[IBIS Ver]   3.2
[File Name]   sprm456.ibs
[File Rev]   1.0
[Date]   November 3, 2003
[Source]   File originated at Texas Instruments
[Copyright]   (c) 2003, Texas Instruments Inc.
[Component]   r2812pgf
[Manufacturer] Texas Instruments
[Package]
| Variable   Typ   Min   Max
R_pkg   0.198   0.1909   0.2047
L_pkg   8.904e-09   8.346e-09   9.905e-09
C_pkg   1.561e-12   1.156e-12   1.834e-12
[Pin] signal_name   model_name   R_pin   L_pin   C_pin
1   VDDAIO   NC   0.1921  9.905e-09  1.489e-12
2   ADCINB0   NC   0.1951  9.662e-09  1.834e-12
3   ADCINB1   NC   0.198   9.558e-09  1.805e-12
4   ADCINB2   NC   0.2006  9.473e-09  1.771e-12
5   ADCINB3   NC   0.2031  9.41e-09   1.706e-12
6   ADCINB4   NC   0.2036  9.308e-09  1.669e-12
7   ADCINB5   NC   0.2017  9.182e-09  1.673e-12
8   ADCINB6   NC   0.2002  9.071e-09  1.647e-12
9   ADCINB7   NC   0.1989  8.977e-09  1.625e-12
10   ADCREFM   NC   0.1977  8.88e-09   1.606e-12
11   ADCREFP   NC   0.1967  8.794e-09  1.581e-12
12   AVSSREFBG   NC   0.1961  8.721e-09  1.56e-12
13   AVDDREFBG   NC   0.1955  8.646e-09  1.544e-12
14   VDDA1   NC   0.195   8.579e-09  1.521e-12
15   VSSA1   NC   0.1949  8.524e-09  1.503e-12
16   ADCRESEXT   NC   0.1948  8.469e-09  1.489e-12
17   XMPNMC   IDG09_PE100   0.1948  8.424e-09  1.468e-12
18   XA(0)   OUI83   0.1952  8.388e-09  1.452e-12
19   VSS   NC   0.1954  8.359e-09  1.442e-12
20   MDRA   IDG09_OUO43_PS100 0.196   8.346e-09  1.424e-12
21   XD(0)   IDG09_OUI83_PS100 0.1967  8.36e-09   1.411e-12
22   MDXA   IDG09_OUO43   0.1975  8.421e-09  1.16e-12
23   VDD   NC   0.198   8.429e-09  1.156e-12
24   XD(1)   IDG09_OUI83_PS100  0.1973  8.376e-09  1.412e-12
25   MCLKRA   IDG09_OUO43_PS100 0.1971  8.373e-09  1.43e-12
26   MFSXA   IDG09_OUO43_PS100 0.197   8.398e-09  1.442e-12
27   XD(2)   IDG09_OUI83_PS100 0.197   8.435e-09  1.457e-12
28   MCLKXA   IDG09_OUO43_PS100 0.1974  8.484e-09  1.476e-12
29   MFSRA   IDG09_OUO43_PS100 0.1977  8.542e-09  1.493e-12
30   XD(3)   IDG09_OUI83_PS100 0.1984  8.61e-09   1.5e-12
31   VDDIO   NC   0.1982  8.656e-09  1.517e-12
32   VSS   NC   0.1989  8.731e-09  1.548e-12
33   XD(4)   IDG09_OUI83_PS100 0.2001  8.817e-09  1.558e-12
34   SPICLKA   IDG09_OUO43   0.1999  8.873e-09  1.577e-12
35   SPISTEA   IDG09_OUO43   0.2013  8.967e-09  1.609e-12
36   XD(5)   IDG09_OUI83_PS100 0.2027  9.071e-09  1.622e-12
37   VDD   NC   0.2027  9.139e-09  1.641e-12
38   VSS   NC   0.2047  9.255e-09  1.665e-12
39   XD(6)   IDG09_OUI83_PS100 0.2047  9.341e-09  1.652e-12
40   SPISIMOA   IDG09_OUO43   0.2031  9.409e-09  1.689e-12
41   SPISOMIA   IDG09_OUO43   0.1983  9.422e-09  1.757e-12
42   XRDn   OUI83   0.1956  9.501e-09  1.801e-12
43   XA(1)   OUI83   0.1933  9.619e-09  1.832e-12
44   XZCS0AND1n   OUI83   0.1909  9.876e-09  1.489e-12
45   PWM7   IDG09_OUO43_PS100 0.1921  9.905e-09  1.489e-12
46   PWM8   IDG09_OUO43_PS100 0.1951  9.662e-09  1.834e-12
47   PWM9   IDG09_OUO43_PS100 0.198   9.558e-09  1.805e-12
48   PWM10   IDG09_OUO43_PS100 0.2006  9.473e-09  1.771e-12
49   PWM11   IDG09_OUO43_PS100 0.2031  9.41e-09   1.706e-12
50   PWM12   IDG09_OUO43_PS100 0.2036  9.308e-09  1.669e-12
51   XRNW   OUI83   0.2017  9.182e-09  1.673e-12
52   VSS   NC   0.2002  9.071e-09  1.647e-12
53   T3PWM_T3CMP   IDG09_OUO43_PS100 0.1989  8.977e-09  1.625e-12
54   XD(7)   IDG09_OUI83_PS100 0.1977  8.88e-09   1.606e-12
55   T4PWM_T4CMP   IDG09_OUO43_PS100 0.1967  8.794e-09  1.581e-12
56   VDD   NC   0.1961  8.721e-09  1.56e-12
57   CAP4_QEP3   IDG09_OUO43_PS100 0.1955  8.646e-09  1.544e-12
58   VSS   NC   0.195   8.579e-09  1.521e-12
59   CAP5_QEP4   IDG09_OUO43_PS100 0.1949  8.524e-09  1.503e-12
60   CAP6_QEPI2   IDG09_OUO43_PS100 0.1948  8.469e-09  1.489e-12
61   C4TRIPn   IDG09_OUO43_PS100 0.1948  8.424e-09  1.468e-12
62   C5TRIPn   IDG09_OUO43_PS100 0.1952  8.388e-09  1.452e-12
63   C6TRIPn   IDG09_OUO43_PS100 0.1954  8.359e-09  1.442e-12
64   VDDIO   NC   0.196   8.346e-09  1.424e-12
65   XD(8)   IDG09_OUI83_PS100 0.1967  8.36e-09   1.411e-12
66   TEST2   NC   0.1975  8.421e-09  1.16e-12
67   TEST1   NC   0.198   8.429e-09  1.156e-12
68   XD(9)   IDG09_OUI83_PS100 0.1973  8.376e-09  1.412e-12
69   VDDIO   NC   0.1971  8.373e-09  1.43e-12
70   VSS   NC   0.197   8.398e-09  1.442e-12
71   TDIRB   IDG09_OUO43_PS100 0.197   8.435e-09  1.457e-12
72   TCLKINB   IDG09_OUO43_PS100 0.1974  8.484e-09  1.476e-12
73   XD(10)   IDG09_OUI83_PS100 0.1977  8.542e-09  1.493e-12
74   XD(11)   IDG09_OUI83_PS100 0.1984  8.61e-09   1.5e-12
75   VDD   NC   0.1982  8.656e-09  1.517e-12
76   X2   NC   0.1989  8.731e-09  1.548e-12
77   X1/XCLKIN   NC   0.2001  8.817e-09  1.558e-12
78   VSS   NC   0.1999  8.873e-09  1.577e-12
79   T3CTRIP_PDPINTBn IDG09_OUO43_PS100 0.2013  8.967e-09  1.609e-12
80   XA(2)   OUI83   0.2027  9.071e-09  1.622e-12
81   VDDIO   NC   0.2027  9.139e-09  1.641e-12
82   XHOLDAn   OUI83   0.2047  9.255e-09  1.665e-12
83   T4CTRIPn/EVBSOCn IDG09_OUO43_PS100 0.2047  9.341e-09  1.652e-12
84   XWEn   OUI83   0.2031  9.409e-09  1.689e-12
85   XA(3)   OUI83   0.1983  9.422e-09  1.757e-12
86   VSS   NC   0.1956  9.501e-09  1.801e-12
87   CANTXA   IDG09_OUO43_PS100 0.1933  9.619e-09  1.832e-12
88   XZCS2n   OUI83   0.1909  9.876e-09  1.489e-12
89   CANRXA   IDG09_OUO43_PS100 0.1921  9.905e-09  1.489e-12
90   SCITXDB   IDG09_OUO43   0.1951  9.662e-09  1.834e-12
91   SCIRXDB   IDG09_OUO43   0.198   9.558e-09  1.805e-12
92   PWM1   IDG09_OUO43_PS100 0.2006  9.473e-09  1.771e-12
93   PWM2   IDG09_OUO43_PS100 0.2031  9.41e-09   1.706e-12
94  PWM3   IDG09_OUO43_PS100  0.2036  9.308e-09  1.669e-12
95   PWM4   IDG09_OUO43_PS100 0.2017  9.182e-09  1.673e-12
96   XD(12)   IDG09_OUI83_PS100 0.2002  9.071e-09  1.647e-12
97   XD(13)   IDG09_OUI83_PS100 0.1989  8.977e-09  1.625e-12
98   PWM5   IDG09_OUO43_PS100 0.1977  8.88e-09   1.606e-12
99   VSS   NC   0.1967  8.794e-09  1.581e-12
100   VDD   NC   0.1961  8.721e-09  1.56e-12
101   PWM6   IDG09_OUO43_PS100 0.1955  8.646e-09  1.544e-12
102   T1PWM_T1CMP   IDG09_OUO43_PS100 0.195   8.579e-09  1.521e-12
103   XA(4)   OUI83   0.1949  8.524e-09  1.503e-12
104   T2PWM_T2CMP   IDG09_OUO43_PS100 0.1948  8.469e-09  1.489e-12
105   VSS   NC   0.1948  8.424e-09  1.468e-12
106   CAP1_QEP1   IDG09_OUO43_PS100 0.1952  8.388e-09  1.452e-12
107   CAP2_QEP2   IDG09_OUO43_PS100 0.1954  8.359e-09  1.442e-12
108   XA(5)   OUI83   0.196   8.346e-09  1.424e-12
109   CAP3_QEPI1   IDG09_OUO43_PS100  0.1967  8.36e-09   1.411e-12
110   T1CTRIP_PDPINTAn IDG09_OUO43_PS100 0.1975  8.421e-09  1.16e-12
111   XA(6)   OUI83   0.198   8.429e-09  1.156e-12
112   VDD   NC   0.1973  8.376e-09  1.412e-12
113   VSS   NC   0.1971  8.373e-09  1.43e-12
114   VDDIO   NC   0.197   8.398e-09  1.442e-12
115   T2CTRIPn/EVASOCn IDG09_OUO43_PS100 0.197   8.435e-09  1.457e-12
116   TDIRA   IDG09_OUO43_PS100 0.1974  8.484e-09  1.476e-12
117   TCLKINA   IDG09_OUO43_PS100 0.1977  8.542e-09  1.493e-12
118   XA(7)   OUI83   0.1984  8.61e-09   1.5e-12
119   XCLKOUT   OUI83   0.1982  8.656e-09  1.517e-12
120   VSS   NC   0.1989  8.731e-09  1.548e-12
121   XA(8)   OUI83   0.2001  8.817e-09  1.558e-12
122   C1TRIPn   IDG09_OUO43_PS100 0.1999  8.873e-09  1.577e-12
123   C2TRIPn   IDG09_OUO43_PS100 0.2013  8.967e-09  1.609e-12
124   C3TRIPn   IDG09_OUO43_PS100 0.2027  9.071e-09  1.622e-12
125   XA(9)   OUI83   0.2027  9.139e-09  1.641e-12
126   TMS   IDG09_PS100   0.2047  9.255e-09  1.665e-12
127   TDO   OUI83   0.2047  9.341e-09  1.652e-12
128   VDD   NC   0.2031  9.409e-09  1.689e-12
129   VSS   NC   0.1983  9.422e-09  1.757e-12
130   XA(10)   OUI83   0.1956  9.501e-09  1.801e-12
131   TDI   IDG09_PS100   0.1933  9.619e-09  1.832e-12
132   XA(11)   OUI83   0.1909  9.876e-09  1.489e-12
133   XZCS6AND7n   OUI83   0.1921  9.905e-09  1.489e-12
134   TESTSEL   IDG09_PE100   0.1951  9.662e-09  1.834e-12
135   TRSTn   IDG09_PE100   0.198   9.558e-09  1.805e-12
136   TCK   IDG09_PS100   0.2006  9.473e-09  1.771e-12
137   EMU0   IDG09_OUI83_PS100 0.2031  9.41e-09   1.706e-12
138   XA(12)   OUI83   0.2036  9.308e-09  1.669e-12
139   XD(14)   IDG09_OUI83_PS100 0.2017  9.182e-09  1.673e-12
140   XF_XPLLDIS   IDG09_OUI83_PS100 0.2002  9.071e-09  1.647e-12
141   XA(13)   OUI83   0.1989  8.977e-09  1.625e-12
142   VSS   NC   0.1977  8.88e-09   1.606e-12
143   VDD   NC   0.1967  8.794e-09  1.581e-12
144   XA(14)   OUI83   0.1961  8.721e-09  1.56e-12
145   VDDIO   NC   0.1955  8.646e-09  1.544e-12
146   EMU1   IDG09_OUI83_PS100  0.195   8.579e-09  1.521e-12
147   XD(15)   IDG09_OUI83_PS100 0.1949  8.524e-09  1.503e-12
148   XA(15)   OUI83   0.1948  8.469e-09  1.489e-12
149   XINT1_XBIOn   IDG09_OUO43   0.1948  8.424e-09  1.468e-12
150   XNMI_XINT13   IDG09_OUO43_PS100 0.1952  8.388e-09  1.452e-12
151   XINT2_ADCSOC   IDG09_OUO43   0.1954  8.359e-09  1.442e-12
152   XA(16)   OUI83   0.196   8.346e-09  1.424e-12
153   VSS   NC   0.1967  8.36e-09   1.411e-12
154   VDD   NC   0.1975  8.421e-09  1.16e-12
155   SCITXDA   IDG09_OUO43_PS100 0.198   8.429e-09  1.156e-12
156   XA(17)   OUI83   0.1973  8.376e-09  1.412e-12
157   SCIRXDA   IDG09_OUO43_PS100 0.1971  8.373e-09  1.43e-12
158   XA(18)   OUI83   0.197   8.398e-09  1.442e-12
159   XHOLDn   IDG09_PS100   0.197   8.435e-09  1.457e-12
160   XRSn   IDG09_OUM42_PS100 0.1974  8.484e-09  1.476e-12
161   XREADY   IDG09_PS100   0.1977  8.542e-09  1.493e-12
162   VDD1   NC   0.1984  8.61e-09   1.5e-12
163   VSS1   NC   0.1982  8.656e-09  1.517e-12
164   ADCBGREFIN   NC   0.1989  8.731e-09  1.548e-12
165   VSSA2   NC   0.2001  8.817e-09  1.558e-12
166   VDDA2   NC   0.1999  8.873e-09  1.577e-12
167   ADCINA7   NC   0.2013  8.967e-09  1.609e-12
168   ADCINA6   NC   0.2027  9.071e-09  1.622e-12
169   ADCINA5   NC   0.2027  9.139e-09  1.641e-12
170   ADCINA4   NC   0.2047  9.255e-09  1.665e-12
171   ADCINA3   NC   0.2047  9.341e-09  1.652e-12
172   ADCINA2   NC   0.2031  9.409e-09  1.689e-12
173   ADCINA1   NC   0.1983  9.422e-09  1.757e-12
174   ADCINA0   NC   0.1956  9.501e-09  1.801e-12
175   ADCLO   NC   0.1933  9.619e-09  1.832e-12
176   VSSAIO   NC   0.1909  9.876e-09  1.489e-12
| End of package information
|   GS30 Cell IDG09_PE100
|   Component IDG09_PE100
[Component]   IDG09_PE100
[Manufacturer]   Texas Instruments
[Package]
|  variable   typ   min   max
R_pkg   0   0   0
L_pkg   0   0   0
C_pkg   0   0   0
[Pin]   signal_name   model_name   R_pin   L_pin   C_pin
VDDS   VDDS   POWER
VSS   VSS   GND
PAD   PAD   IDG09_PE100
[Model Selector] IDG09_PE100
9_PE100_PULLDOWN_2P5  Cell operated at 2.5(nom)
|IDG09_PE100_PULLDOWN_2P5; BUFFER WITH WEAK_PULLDOWN_ON
PE100_NOPULLDOWN_2P5  Cell operated at 2.5(nom)
|IDG09_PE100_NOPULLDOWN_2P5; BUFFER OPERATING IN NORMMAL MODE WITHOUT PULLD
|OWN
9_PE100_PULLDOWN_3P3  Cell operated at 3.3(nom)
|IDG09_PE100_PULLDOWN_3P3; BUFFER WITH WEAK_PULLDOWN_ON
PE100_NOPULLDOWN_3P3  Cell operated at 3.3(nom)
|IDG09_PE100_NOPULLDOWN_3P3; BUFFER OPERATING IN NORMMAL MODE WITHOUT PULLD
|OWN
_PE100_PULLDOWN_2P75  Cell operated at 2.75(nom)
|IDG09_PE100_PULLDOWN_2P75; BUFFER WITH WEAK_PULLDOWN_ON
E100_NOPULLDOWN_2P75  Cell operated at 2.75(nom)
[Component]   IDG09_OUO43
[Manufacturer]   Texas Instruments
[Package]
|  variable   typ   min   max
R_pkg   0   0   0
L_pkg   0   0   0
C_pkg   0   0   0
[Pin]   signal_name   model_name   R_pin   L_pin   C_pin
VSS   VSS   GND
VDDS   VDDS   POWER
PAD   PAD   IDG09_OUO43
[Model Selector] IDG09_OUO43
IDG09_OUO43_2P5  Cell operated at 2.5(nom)
|IDG09_OUO43_2P5; DEFAULT
IDG09_OUO43_3P3  Cell operated at 3.3(nom)
|IDG09_OUO43_3P3; DEFAULT
IDG09_OUO43_2P75  Cell operated at 2.75(nom)
|   Component IDG09_PS100
[Component]   IDG09_PS100
[Manufacturer]   Texas Instruments
[Package]
|  variable   typ   min   max
R_pkg   0   0   0
L_pkg   0   0   0
C_pkg   0   0   0
[Pin]   signal_name   model_name   R_pin   L_pin   C_pin
VDDS   VDDS   POWER
VSS   VSS   GND
PAD   PAD   IDG09_PS100
[Model Selector] IDG09_PS100
G09_PS100_PULLUP_2P5  Cell operated at 2.5(nom)
|IDG09_PS100_PULLUP_2P5; BUFFER WITH WEAK_PULLUP_ON
9_PS100_NOPULLUP_2P5  Cell operated at 2.5(nom)
|IDG09_PS100_NOPULLUP_2P5; BUFFER OPERATING IN NORMMAL MODE WITHOUT PULLUP
G09_PS100_PULLUP_3P3  Cell operated at 3.3(nom)
|IDG09_PS100_PULLUP_3P3; BUFFER WITH WEAK_PULLUP_ON
9_PS100_NOPULLUP_3P3  Cell operated at 3.3(nom)
|IDG09_PS100_NOPULLUP_3P3; BUFFER OPERATING IN NORMMAL MODE WITHOUT PULLUP
09_PS100_PULLUP_2P75  Cell operated at 2.75(nom)
|IDG09_PS100_PULLUP_2P75; BUFFER WITH WEAK_PULLUP_ON
_PS100_NOPULLUP_2P75  Cell operated at 2.75(nom)
|   Component OUI83
[Component]   OUI83
[Manufacturer]   Texas Instruments
[Package]
|  variable   typ   min   max
R_pkg   0   0   0
L_pkg   0   0   0
C_pkg   0   0   0
[Pin]   signal_name   model_name   R_pin   L_pin   C_pin
VSS   VSS   GND
VDDS   VDDS   POWER
Y   Y   OUI83
[Model Selector] OUI83
OUI83_2P5  Cell operated at 2.5(nom)
|OUI83_2P5; DEFAULT
OUI83_3P3  Cell operated at 3.3(nom)
|OUI83_3P3; DEFAULT
OUI83_2P75  Cell operated at 2.75(nom)
|   Component IDG09_OUI83_PS100
[Component]   IDG09_OUI83_PS100
[Manufacturer]   Texas Instruments
[Package]
|  variable   typ   min   max
R_pkg   0   0   0
L_pkg   0   0   0
C_pkg   0   0   0
[Pin]   signal_name   model_name   R_pin   L_pin   C_pin
VSS   VSS   GND
VDDS   VDDS   POWER
PAD   PAD   IDG09_OUI83_PS100
[Model Selector] IDG09_OUI83_PS100
UI83_PS100_PU_ON_2P5  Cell operated at 2.5(nom)
|IDG09_OUI83_PS100_PU_ON_2P5; BUFFER WITH WEAK_PULLUP_ON
I83_PS100_PU_OFF_2P5  Cell operated at 2.5(nom)
|IDG09_OUI83_PS100_PU_OFF_2P5; BUFFER IN NORMAL MODE WITH PULLUP AND PUL
|LDOWN OFF
UI83_PS100_PU_ON_3P3  Cell operated at 3.3(nom)
|IDG09_OUI83_PS100_PU_ON_3P3; BUFFER WITH WEAK_PULLUP_ON
I83_PS100_PU_OFF_3P3  Cell operated at 3.3(nom)
|IDG09_OUI83_PS100_PU_OFF_3P3; BUFFER IN NORMAL MODE WITH PULLUP AND PUL
|LDOWN OFF
I83_PS100_PU_ON_2P75  Cell operated at 2.75(nom)
|IDG09_OUI83_PS100_PU_ON_2P75; BUFFER WITH WEAK_PULLUP_ON
83_PS100_PU_OFF_2P75  Cell operated at 2.75(nom)
|   Component IDG09_OUO43_PS100
[Component]   IDG09_OUO43_PS100
[Manufacturer]   Texas Instruments
[Package]
|  variable   typ   min   max
R_pkg   0   0   0
L_pkg   0   0   0
C_pkg   0   0   0
[Pin]   signal_name   model_name   R_pin   L_pin   C_pin
VSS   VSS   GND
VDDS   VDDS   POWER
PAD   PAD   IDG09_OUO43_PS100
[Model Selector] IDG09_OUO43_PS100
UO43_PS100_PU_ON_2P5  Cell operated at 2.5(nom)
|IDG09_OUO43_PS100_PU_ON_2P5; BUFFER WITH WEAK_PULLUP_ON
O43_PS100_PU_OFF_2P5  Cell operated at 2.5(nom)
|IDG09_OUO43O43_PS100_PU_OFF_2P5; BUFFER IN NORMAL MODE WITH PULLUP
| OFF
UO43_PS100_PU_ON_3P3  Cell operated at 3.3(nom)
|IDG09_OUO43_PS100_PU_ON_3P3; BUFFER WITH WEAK_PULLUP_ON
O43_PS100_PU_OFF_3P3  Cell operated at 3.3(nom)
|IDG09_OUO43_PS100_PU_OFF_3P3; BUFFER IN NORMAL MODE WITH PULLUP
| OFF
O43_PS100_PU_ON_2P75  Cell operated at 2.75(nom)
|IDG09_OUO43_PS100_PU_ON_2P75; BUFFER WITH WEAK_PULLUP_ON
43_PS100_PU_OFF_2P75  Cell operated at 2.75(nom)
|   Component IDG09_OUM42_PS100
[Component]   IDG09_OUM42_PS100
[Manufacturer]   Texas Instruments
[Package]
|  variable   typ   min   max
R_pkg   0   0   0
L_pkg   0   0   0
C_pkg   0   0   0
[Pin]   signal_name   model_name   R_pin   L_pin   C_pin
VSS   VSS   GND
VDDS   VDDS   POWER
PAD   PAD   IDG09_OUM42_PS100
[Model Selector] IDG09_OUM42_PS100
UM42_PS100_PU_ON_2P5  Cell operated at 2.5(nom)
|IDG09_OUM42_PS100_PU_ON_2P5; BUFFER WITH WEAK_PULLUP_ON
M42_PS100_PU_OFF_2P5  Cell operated at 2.5(nom)
|IDG09_OUM42_PS100_PU_OFF_2P5; BUFFER IN NORMAL MODE WITH PULLUP OFF
UM42_PS100_PU_ON_3P3  Cell operated at 3.3(nom)
|IDG09_OUM42_PS100_PU_ON_3P3; BUFFER WITH WEAK_PULLUP_ON
M42_PS100_PU_OFF_3P3  Cell operated at 3.3(nom)
|IDG09_OUM42_PS100_PU_OFF_3P3; BUFFER IN NORMAL MODE WITH PULLUP OFF
M42_PS100_PU_ON_2P75  Cell operated at 2.75(nom)
|IDG09_OUM42_PS100_PU_ON_2P75; BUFFER WITH WEAK_PULLUP_ON
42_PS100_PU_OFF_2P75  Cell operated at 2.75(nom)
| Models and submodels in the file (36): 9_PE100_PULLDOWN_2P5 (Input), PE100_NOPULLDOWN_2P5 (Input), 9_PE100_PULLDOWN_3P3 (Input), PE100_NOPULLDOWN_3P3 (Input), _PE100_PULLDOWN_2P75 (Input), E100_NOPULLDOWN_2P75 (Input), IDG09_OUO43_2P5 (I/O), IDG09_OUO43_3P3 (I/O), IDG09_OUO43_2P75 (I/O), G09_PS100_PULLUP_2P5 (Input), 9_PS100_NOPULLUP_2P5 (Input), G09_PS100_PULLUP_3P3 (Input), 9_PS100_NOPULLUP_3P3 (Input), 09_PS100_PULLUP_2P75 (Input), _PS100_NOPULLUP_2P75 (Input), OUI83_2P5 (3-state), OUI83_3P3 (3-state), OUI83_2P75 (3-state), UI83_PS100_PU_ON_2P5 (I/O), I83_PS100_PU_OFF_2P5 (I/O), UI83_PS100_PU_ON_3P3 (I/O), I83_PS100_PU_OFF_3P3 (I/O), I83_PS100_PU_ON_2P75 (I/O), 83_PS100_PU_OFF_2P75 (I/O), UO43_PS100_PU_ON_2P5 (I/O), O43_PS100_PU_OFF_2P5 (I/O), UO43_PS100_PU_ON_3P3 (I/O), O43_PS100_PU_OFF_3P3 (I/O), O43_PS100_PU_ON_2P75 (I/O), 43_PS100_PU_OFF_2P75 (I/O), UM42_PS100_PU_ON_2P5 (I/O_open_drain), M42_PS100_PU_OFF_2P5 (I/O_open_drain), UM42_PS100_PU_ON_3P3 (I/O_open_drain), M42_PS100_PU_OFF_3P3 (I/O_open_drain), M42_PS100_PU_ON_2P75 (I/O_open_drain), 42_PS100_PU_OFF_2P75 (I/O_open_drain)
